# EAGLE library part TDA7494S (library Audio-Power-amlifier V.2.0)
The TDA7494S 10W is class AB power amplifier assembled in the @Multiwatt 15 package, specially designed for high quality sound, TV applications. Features of the TDA7494S include Stand-by and mute functions.
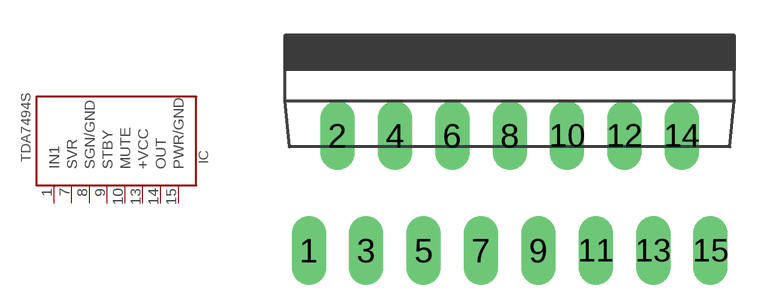
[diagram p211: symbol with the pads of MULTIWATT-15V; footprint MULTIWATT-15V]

Designator prefix IC

## TDA7494S  [MULTIWATT-15V]
1  IN1  in
7  SVR  in
8  SGN/GND  pwr
9  STBY  in
10  MUTE  in
13  +VCC  pwr
14  OUT  out
15  PWR/GND  pwr

## Footprint MULTIWATT-15V (pad centres in mm)
Multiwatt 15 vertical
drill 1.016 long: 1 -8.89,-5.08; 2 -7.62,0; 3 -6.35,-5.08; 4 -5.08,0; 5 -3.81,-5.08; 6 -2.54,0; 7 -1.27,-5.08; 8 0,0; 9 1.27,-5.08; 10 2.54,0; 11 3.81,-5.08; 12 5.08,0; 13 6.35,-5.08; 14 7.62,0; 15 8.89,-5.08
